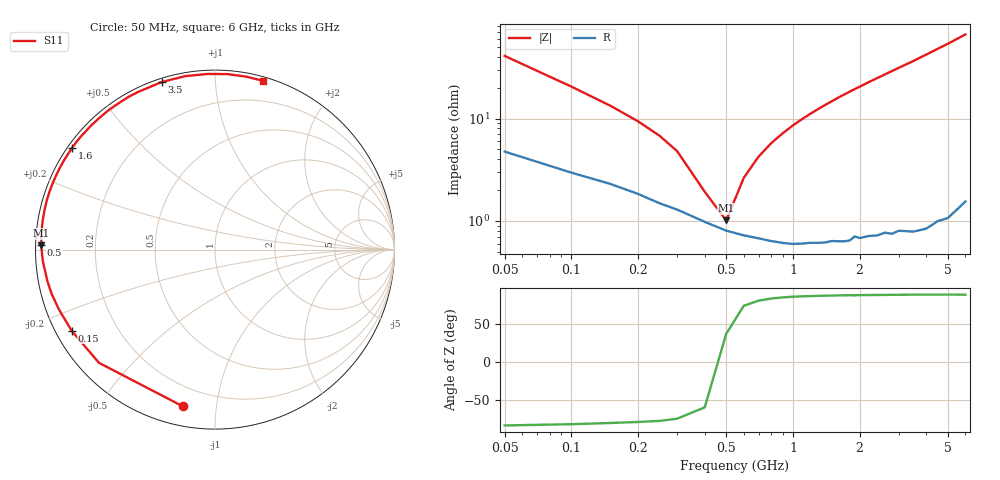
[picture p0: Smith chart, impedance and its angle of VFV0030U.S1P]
! Infineon Technologies  Discrete & RF Semiconductors
! BBY 58-03
! Si Tuning Diode in SOD323
! VR =
! S-Parameters:  June  1999
# GHz  S  MA  R  50
!  f  S11
! GHz  MAG  ANG
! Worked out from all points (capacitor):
!   34 points, 50 MHz to 6 GHz, reference 50 ohm
!   read as one part to ground: C = 74.9 pF near 50 MHz
!   lowest |Z| = 1.01 ohm at 500 MHz (marker M1)
!   series resonance near 473.1 MHz, so ESL is about 1.5 nH
!   S11 on the Smith chart (normalised r, x): 50 MHz: 0.10, -0.81; 150 MHz: 0.05, -0.26; 500 MHz: 0.02, +0.01; 1.6 GHz: 0.01, +0.32; 3.5 GHz: 0.02, +0.73; 6 GHz: 0.03, +1.32
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0.05  0.8919 -101.5
0.1  0.9033 -135.7
0.15  0.9176 -150.5
0.2  0.9315 -159.1
0.25  0.9432 -164.9
0.3  0.9501 -169.4
0.4  0.9617 -176.2
0.5  0.9684 178.6
0.6  0.9716 174.2
0.7  0.9735 170.4
0.8  0.9752 166.9
1  0.9771 160.6
1.2  0.977 154.9
1.4  0.9773 149.6
1.6  0.9773 144.6
1.8  0.9776 139.9
2  0.977 135.5
2.2  0.9767 131.2
2.4  0.9771 127.2
2.6  0.9765 123.3
2.8  0.9779 119.6
3  0.9772 116.0
3.5  0.9797 107.7
4  0.9805 99.7
4.5  0.9795 92.4
5  0.9804 85.9
5.5  0.979 79.6
6  0.9778 74.1
